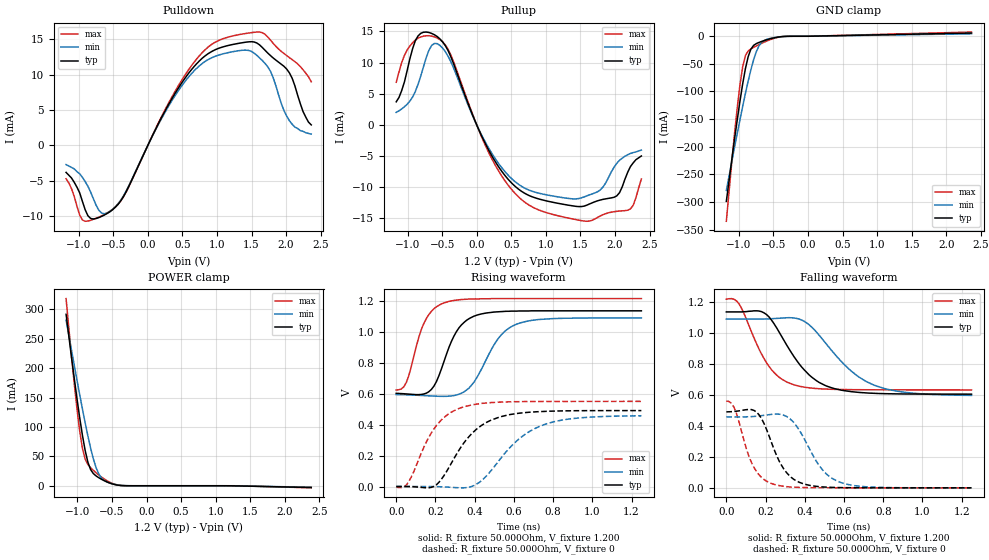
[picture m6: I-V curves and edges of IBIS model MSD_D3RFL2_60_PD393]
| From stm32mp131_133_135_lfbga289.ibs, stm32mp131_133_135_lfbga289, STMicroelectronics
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[Model] MSD_D3RFL2_60_PD393
Model_type   I/O
C_comp 2.371pF   2.287pF   2.495pF
Vinh = 820.000mV
Vinl = 380.000mV
Vmeas = 600.000mV
Vref = 600.000mV
[Model Spec]
Vinh   820.000mV   790.000mV   870.000mV
Vinl   380.000mV   350.000mV   430.000mV
Vmeas   600.000mV   570.000mV   650.000mV
Vref   600.000mV   570.000mV   650.000mV
[Receiver Thresholds]
Vth   =  0.600V
Vth_min  =  0.5880V
Vth_max  =  0.6120V
Vinh_ac  =  0.220V
Vinh_dc  =  0.130V
Vinl_ac  = -0.220V
Vinl_dc  = -0.130V
Tslew_ac =  5.000ns |Not specified, so set to high value
[Temperature Range]   25.000   125.000   -40.000
[Voltage Range]   1.200V   1.140V   1.300V
[GND Clamp Reference]   0.00V   0.00V   0.00V
[Pulldown Reference]   0.00V   0.00V   0.00V
[POWER Clamp Reference]   1.200V   1.140V   1.300V
[Pullup Reference]   1.200V   1.140V   1.300V
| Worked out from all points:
|   slope of the pulldown table from 0 to 0.18 V, typ, clamps not added: 50.1 ohm
|   slope of the pullup table from 0 to 0.18 V, typ, clamps not added: 42.9 ohm
|   GND clamp passes 1 mA (typ) near -0.40 V on its own axis
|   POWER clamp passes 1 mA (typ) near -0.42 V on its own axis
|   rising waveform, R_fixture 50.000Ohm, V_fixture 1.200: 20-80 % time 107ps typ, 138ps min, 89.2ps max; typ from 0.603 V to 1.14 V
|   rising waveform, R_fixture 50.000Ohm, V_fixture 0: 20-80 % time 175ps typ, 217ps min, 145ps max; typ from 0.001 V to 0.492 V
|   falling waveform, R_fixture 50.000Ohm, V_fixture 1.200: 20-80 % time 181ps typ, 232ps min, 142ps max; typ from 1.14 V to 0.606 V
|   falling waveform, R_fixture 50.000Ohm, V_fixture 0: 20-80 % time 107ps typ, 134ps min, 91.3ps max; typ from 0.491 V to 0 V
[GND Clamp]
-1.182V   -298.9mA   -279mA     -334.9mA
-1.064V   -186.7mA   -201.4mA   -176.7mA
-984.9mV  -117.4mA   -151.2mA   -87.93mA
-945.5mV  -86.07mA   -127mA     -55.15mA
-906.1mV  -58.69mA   -103.6mA   -35.07mA
-866.7mV  -37.21mA   -81.39mA   -26.69mA
-787.9mV  -16.61mA   -42.71mA   -20.15mA
-709.1mV  -11.16mA   -17.31mA   -15.09mA
-630.3mV  -7.681mA   -7.385mA   -10.44mA
-512.1mV  -3.463mA   -2.956mA   -4.587mA
-315.1mV  -156.4uA   -222.4uA   -144.7uA
2.364V    5.825mA    4.473mA    7.624mA
[Power Clamp]
-1.164V   291.7mA    281.8mA    318.4mA
-1.085V   218mA      230.2mA    219.3mA
-1.006V   147.9mA    179.5mA    130.4mA
-966.7mV  115.4mA    154.7mA    92.71mA
-927.3mV  85.63mA    130.4mA    63.4mA
-887.9mV  59.94mA    106.9mA    45.32mA
-809.1mV  27.44mA    63.95mA    30.69mA
-730.3mV  16.73mA    30.86mA    22.05mA
-690.9mV  13.67mA    20.06mA    18.23mA
-572.7mV  6.475mA    6.385mA    8.584mA
-336.4mV  171uA      329.6uA    200.9uA
2.382V    -2.997mA   -2.472mA   -3.554mA
[Pulldown]
-1.182V   -3.8mA     -2.7mA     -4.7mA
-945.5mV  -7.9mA     -4.5mA     -10.52mA
-827.3mV  -10.3mA    -6.57mA    -10.57mA
-669.7mV  -10.02mA   -9.53mA    -9.94mA
-551.5mV  -9.376mA   -9.343mA   -9.301mA
-315.1mV  -6.567mA   -6.464mA   -6.607mA
551.5mV   9.678mA    9.201mA    10.13mA
906.1mV   13.16mA    12.3mA     14.14mA
1.3V      14.39mA    13.36mA    15.61mA
1.733V    13.06mA    11.13mA    15.34mA
2.009V    10.78mA    4.14mA     12.69mA
2.364V    2.9mA      1.6mA      9mA
[Pullup]
-1.164V   3.7mA      2.005mA    6.838mA
-1.045V   6.9mA      2.909mA    11.16mA
-887.9mV  13.51mA    5.344mA    13.62mA
-690.9mV  14.84mA    11.98mA    14.32mA
-454.5mV  12.73mA    11.77mA    12.85mA
175.8mV   -4.107mA   -3.772mA   -4.491mA
687.9mV   -10.95mA   -10.12mA   -12.36mA
1.476V    -13.13mA   -11.84mA   -15.31mA
1.791V    -12.06mA   -10.42mA   -14.61mA
1.988V    -11.63mA   -6.789mA   -13.95mA
2.224V    -6.7mA     -4.595mA   -13.49mA
2.382V    -5mA       -4.048mA   -8.7mA
[Ramp]
R_load=50.000Ohm
dV/dt_r   307.140mV/142.000ps  286.469mV/179.000ps  340.320mV/117.000ps
dV/dt_f   307.110mV/146.000ps  286.437mV/185.000ps  340.320mV/116.500ps
[Rising waveform]
R_fixture=50.000Ohm
V_fixture=1.200
V_fixture_min=1.140
V_fixture_max=1.300
0s        603.3mV    595mV      625.1mV
52ps      599.3mV    593.6mV    674.9mV
128ps     596mV      589.6mV    1.016V
166ps     613.4mV    587.1mV    1.112V
243ps     807mV      583.7mV    1.188V
294ps     972.5mV    588.7mV    1.204V
358ps     1.075V     623.9mV    1.212V
524ps     1.131V     963.9mV    1.216V
613ps     1.135V     1.05V      1.216V
1.25ns    1.137V     1.091V     1.216V
[Rising waveform]
R_fixture=50.000Ohm
V_fixture=0
0s        586.5uV    160.5uV    -3.677mV
64ps      189.5uV    511.4uV    31.76mV
192ps     978.4uV    64.61uV    372.3mV
332ps     259mV      -8.025mV   510.7mV
409ps     370.9mV    15.05mV    533.2mV
473ps     423.4mV    87.42mV    542.4mV
600ps     469.8mV    278.6mV    548.9mV
728ps     484.7mV    388mV      550.5mV
894ps     490.3mV    439.1mV    550.9mV
1.25ns    491.6mV    457.8mV    551.2mV
[Falling waveform]
R_fixture=50.000Ohm
V_fixture=1.200
V_fixture_min=1.140
V_fixture_max=1.300
0s        1.137V     1.091V     1.219V
64ps      1.137V     1.091V     1.19V
192ps     1.131V     1.091V     836.6mV
256ps     1.035V     1.095V     729.2mV
332ps     873.2mV    1.099V     671.6mV
409ps     747.1mV    1.066V     648.6mV
498ps     665.3mV    948.2mV    638.8mV
639ps     621.4mV    752.4mV    634.6mV
754ps     610.9mV    663.3mV    633.7mV
1.25ns    605.5mV    597.5mV    632.9mV
[Falling waveform]
R_fixture=50.000Ohm
V_fixture=0
0s        491.1mV    458.4mV    560.9mV
39ps      493.5mV    458.1mV    520.9mV
115ps     506.4mV    459.4mV    204.5mV
154ps     489.6mV    462.8mV    105.1mV
230ps     293.6mV    474.6mV    27.85mV
281ps     146.5mV    474.2mV    11.92mV
345ps     53.88mV    421mV      3.972mV
486ps     6.356mV    123mV      545.5uV
588ps     1.403mV    32.5mV     112.9uV
1.25ns    -1.855uV   4.51uV     -1.824uV
